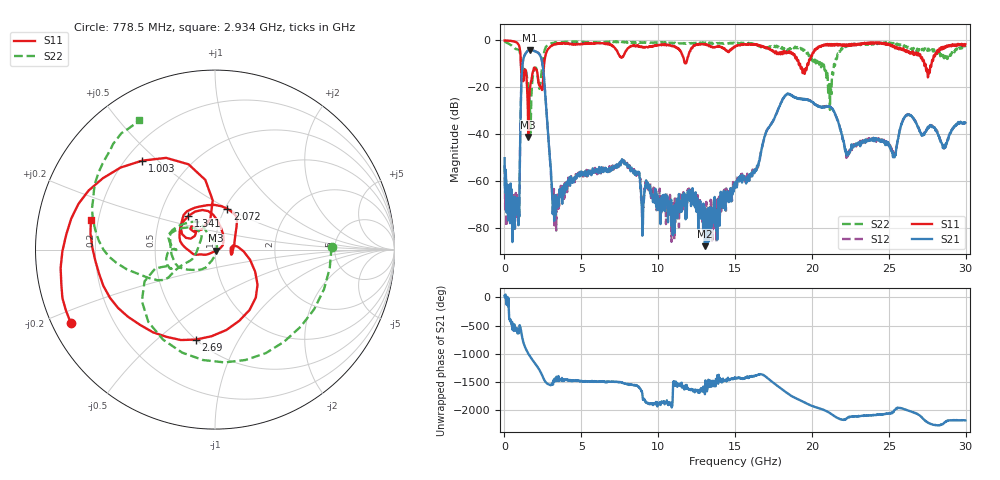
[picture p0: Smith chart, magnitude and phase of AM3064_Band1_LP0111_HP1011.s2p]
# Hz S DB R 50.0
!freq dBS11 angS11 dBS21 angS21 dBS12 angS12 dBS22 angS22
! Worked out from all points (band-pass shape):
!   1600 points, 10 MHz to 29.98 GHz, reference 50 ohm
!   highest |S21| = -4.07 dB at 1.678 GHz (marker M1); lowest = -87.7 dB at 13.04 GHz (marker M2)
!   |S21| within 3 dB of the highest: 1.267 GHz to 2.366 GHz (1.099 GHz wide, 60.5 % of centre)
!   lowest |S11| = -41.1 dB at 1.547 GHz (marker M3), VSWR 1.02, Z = 50.7 - j0.586 ohm
!   |S11| at or under -10 dB: 1.071 GHz to 2.582 GHz (1.511 GHz wide, 82.7 % of centre); 19.22 GHz to 19.71 GHz (481.1 MHz wide, 2.47 % of centre); 27.3 GHz to 27.78 GHz (481.9 MHz wide, 1.75 % of centre)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
!   |S22| runs from -39.5 to -0.4 dB; largest |S21 - S12| = 0.0069
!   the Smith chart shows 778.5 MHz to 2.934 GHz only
!   S11 on the Smith chart (normalised r, x): 778.5 MHz: 0.05, -0.24; 1.003 GHz: 0.27, +0.45; 1.341 GHz: 0.70, +0.28; 2.072 GHz: 1.03, +0.50; 2.69 GHz: 0.50, -0.68; 2.934 GHz: 0.17, +0.11
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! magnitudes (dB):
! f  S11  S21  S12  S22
! 10 MHz  -0.1  -50.2  -53.2  -0.4
! 778.5 MHz  -0.9  -70.5  -71.3  -3.8
! 1.003 GHz  -3.9  -50.8  -50.7  -5.2
! 1.172 GHz  -14.7  -10.4  -10.3  -11.5
! 1.341 GHz  -12.4  -6.0  -5.9  -11.4
! 1.547 GHz  -41.1  -4.3  -4.3  -20.0
! 1.678 GHz  -19.3  -4.1  -4.1  -33.3
! 2.072 GHz  -12.5  -4.9  -4.9  -12.0
! 2.69 GHz  -5.8  -26.3  -26.2  -2.8
! 2.934 GHz  -3.0  -48.1  -47.9  -1.6
! 3.253 GHz  -1.8  -68.8  -78.8  -1.1
! 5.015 GHz  -1.6  -55.9  -57.3  -0.6
! 7.732 GHz  -6.6  -51.8  -51.5  -0.6
! 10 GHz  -2.1  -72.3  -68.1  -0.9
! 13.04 GHz  -1.8  -87.7  -78.5  -1.2
! 15 GHz  -2.8  -63.0  -59.8  -1.4
! 18.25 GHz  -5.0  -23.6  -23.6  -4.2
! 19.99 GHz  -6.7  -26.2  -26.2  -8.0
! 21.17 GHz  -2.0  -28.3  -28.0  -29.6
! 22.32 GHz  -2.0  -48.3  -49.5  -2.5
! 25 GHz  -1.5  -44.4  -44.7  -1.2
! 29.98 GHz  -1.6  -35.1  -35.4  -3.0
